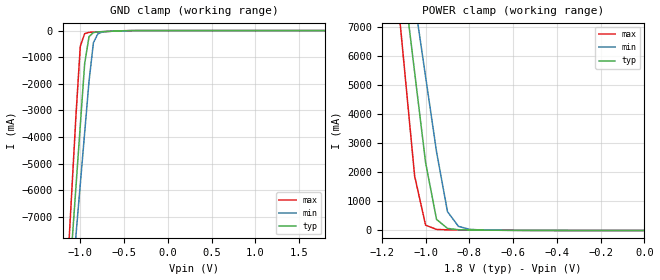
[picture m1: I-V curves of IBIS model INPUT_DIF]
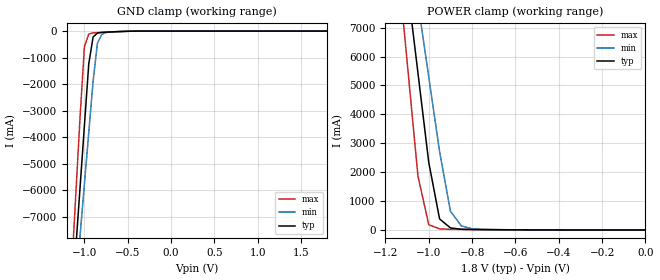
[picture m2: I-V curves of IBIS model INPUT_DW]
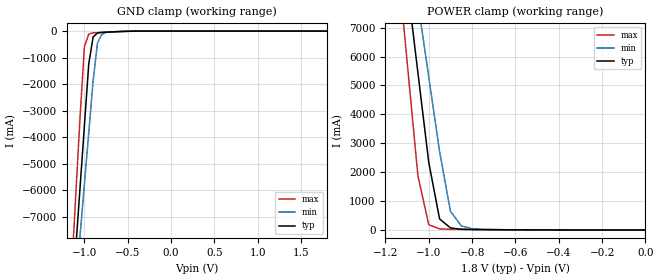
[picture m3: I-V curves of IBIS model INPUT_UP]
|   DIODES INCORPORATED
|   IBIS Model of PI6CB18801
|   Product Family: 6CB
|   TQFN 48-Pins (ZL) Package
[IBIS Ver] 3.2
[Comment char] |_char
[File Name] pi6cb18801_zl_reva.ibs
[File Rev] 1.0
[Source] File originated at Diodes Incorporated.
[Date] 12/18/18
[Disclaimer] (C) Copyright DIODES INCORPORATED
   All rights reserved
  Diodes Incorporated hereby grants the user of
  this IBIS model a non-exclusive, nontransferable license to
  use this IBIS model under the following terms.
  This IBIS model is provided on an "AS IS" basis and Diodes
  makes absolutely no warranty with respect to the information
  contained herein. DIODES DISCLAIMS AND CUSTOMER WAIVES ALL
  WARRANTIES, EXPRESSED OR IMPLIED, INCLUDING WARRANTIES OF
  MERCHANTABILITY OR FITNESS FOR A PARTICULAR PURPOSE. The
  entire risk as to quality and performance is with the customer.
  Accordingly, in no event shall the company be liable for any
  damages, whether in contract or tort, including any lost
  profits or other incidental, consequential, exemplary, or
  punitive damages arising out of the use or application of the
  IBIS model provided in this package. Further, Diodes reserves
  the right to make changes without notice to any product herein
  to improve reliability, function, or design. Diodes does not
  convey any license under patent rights or any other intellectual
  property rights, including those of third parties.
  The user is granted this license only to use the IBIS model
  and is not granted rights to sell, load, rent, lease or license
  the IBIS model in whole or in part, or in modified form to anyone
  other than user. User may modify the IBIS model to suit its specific
  application but rights to derivative works and such modifications
  shall belong to Diodes.
  Diodes is not obligated to provide maintenance or support
  for the licensed IBIS model.
  Contact Diodes at ATTN: APPLICATION ENGINEERING / IBIS MODELS
  1545 Barber Ln. Milpitas, CA 95035
[Component] PI6CB18801
[Manufacturer] Diodes Incorporated.
[Package]
| Variable   typ   min   max
R_pkg   0.03902ohm   0.02922ohm   0.04882ohm
L_pkg   0.79998nH   0.76828nH   0.83168nH
C_pkg   0.19606pF   0.17176pF   0.22036pF
[Pin]  signal_name   model_name   R_pin   L_pin   C_pin
1   SADR_TRI   INPUT_DW   0.04882   0.83168nH   0.22036pF
2   BW_SEL_TRI   NC   0.04490   0.81900nH   0.21064pF
3   NC   NC   0.04098   0.80632nH   0.20092pF
4   NC   NC   0.03706   0.79364nH   0.19120pF
5   VDD_R   POWER   0.03314   0.78096nH   0.18148pF
6   IN+   INPUT_DIF   0.02922   0.76828nH   0.17176pF
7   IN-   INPUT_DIF   0.02922   0.76828nH   0.17176pF
8   GND_R   GND   0.03314   0.78096nH   0.18148pF
9   GND_DIG   GND   0.03706   0.79364nH   0.19120pF
10   SCLK   INPUT_SCLK   0.04098   0.80632nH   0.20092pF
11   SDATA   IO   0.04490   0.81900nH   0.21064pF
12   VDD_DIG   POWER   0.04882   0.83168nH   0.22036pF
13   VDDO   POWER   0.04882   0.83168nH   0.22036pF
14   OE0#   INPUT_DW   0.04490   0.81900nH   0.21064pF
15   Q0+   HCSL_OUT   0.04098   0.80632nH   0.20092pF
16   Q0-   HCSL_OUT   0.03706   0.79364nH   0.19120pF
17   OE1#   INPUT_DW   0.03314   0.78096nH   0.18148pF
18   Q1+   HCSL_OUT   0.02922   0.76828nH   0.17176pF
19   Q1-   HCSL_OUT   0.02922   0.76828nH   0.17176pF
20   VDD   POWER   0.03314   0.78096nH   0.18148pF
21   VDDO   POWER   0.03706   0.79364nH   0.19120pF
22   GND   GND   0.04098   0.80632nH   0.20092pF
23   Q2+   HCSL_OUT   0.04490   0.81900nH   0.21064pF
24   Q2-   HCSL_OUT   0.04882   0.83168nH   0.22036pF
25   OE2#   INPUT_DW   0.04882   0.83168nH   0.22036pF
26   Q3+   HCSL_OUT   0.04490   0.81900nH   0.21064pF
27   Q3-   HCSL_OUT   0.04098   0.80632nH   0.20092pF
28   OE3#   INPUT_DW   0.03706   0.79364nH   0.19120pF
29   GNDA   GND   0.03314   0.78096nH   0.18148pF
30   VDDA   POWER   0.02922   0.76828nH   0.17176pF
31   VDDO   POWER   0.02922   0.76828nH   0.17176pF
32   Q4+   HCSL_OUT   0.03314   0.78096nH   0.18148pF
33   Q4-   HCSL_OUT   0.03706   0.79364nH   0.19120pF
34   OE4#   INPUT_DW   0.04098   0.80632nH   0.20092pF
35   Q5+   HCSL_OUT   0.04490   0.81900nH   0.21064pF
36   Q5-   HCSL_OUT   0.04882   0.83168nH   0.22036pF
37   OE5#   INPUT_DW   0.04882   0.83168nH   0.22036pF
38   VDD   POWER   0.04490   0.81900nH   0.21064pF
39   VDDO   POWER   0.04098   0.80632nH   0.20092pF
40   GND   GND   0.03706   0.79364nH   0.19120pF
41   Q6+   HCSL_OUT   0.03314   0.78096nH   0.18148pF
42   Q6-   HCSL_OUT   0.02922   0.76828nH   0.17176pF
43   OE6#   INPUT_DW   0.02922   0.76828nH   0.17176pF
44   Q7+   HCSL_OUT   0.03314   0.78096nH   0.18148pF
45   Q7-   HCSL_OUT   0.03706   0.79364nH   0.19120pF
46   OE7#   INPUT_DW   0.04098   0.80632nH   0.20092pF
47   VDDO   POWER   0.04490   0.81900nH   0.21064pF
48   PD#   INPUT_UP   0.04882   0.83168nH   0.22036pF
[Diff Pin] inv_pin vdiff  tdelay_typ tdelay_min tdelay_max
15   16   NA   NA   NA   NA
18   19   NA   NA   NA   NA
23   24   NA   NA   NA   NA
26   27   NA   NA   NA   NA
32   33   NA   NA   NA   NA
35   36   NA   NA   NA   NA
41   42   NA   NA   NA   NA
44   45   NA   NA   NA   NA
[Model selector] HCSL_OUT
HCSL_0P6_SLOW  Diff Output,Amplitude=0.6V,SMBUS=2v/ns,slow,slew_rate=0
HCSL_0P6_FAST  Diff Output,Amplitude=0.6V,SMBUS=3v/ns,fast,slew_rate=1
HCSL_0P7_SLOW  Diff Output,Amplitude=0.7V,SMBUS=2v/ns,slow,slew_rate=0
HCSL_0P7_FAST  Diff Output,Amplitude=0.7V,SMBUS=3v/ns,fast,slew_rate=1
HCSL_0P8_SLOW  Diff Output,Amplitude=0.8V,SMBUS=2v/ns,slow,slew_rate=0
HCSL_0P8_FAST  Diff Output,Amplitude=0.8V,SMBUS=3v/ns,fast,slew_rate=1
HCSL_0P9_SLOW  Diff Output,Amplitude=0.9V,SMBUS=2v/ns,slow,slew_rate=0
HCSL_0P9_FAST  Diff Output,Amplitude=0.9V,SMBUS=3v/ns,fast,slew_rate=1
| Models and submodels in the file (13): INPUT_DIF (Input), INPUT_DW (Input), INPUT_UP (Input), INPUT_SCLK (Input), IO (I/O_open_drain), HCSL_0P6_FAST (Output), HCSL_0P6_SLOW (Output), HCSL_0P7_FAST (Output), HCSL_0P7_SLOW (Output), HCSL_0P8_FAST (Output), HCSL_0P8_SLOW (Output), HCSL_0P9_FAST (Output), HCSL_0P9_SLOW (Output)
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|   Model INPUT_DIF
[Model] INPUT_DIF
Model_type Input
Vinl = 540.00mV
Vinh = 1.2600V
| variable   typ   min   max
C_comp   1.000pF   0.997pF   2.003pF
[Voltage Range]   1.8000V   1.7000V   1.9000V
[POWER Clamp Reference]   1.8000V   1.7000V   1.9000V
[GND Clamp Reference]   0.0000V   0.0000V   0.0000V
[Temperature Range]   25   85   -40
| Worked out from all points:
|   GND clamp passes 1 mA (typ) near -0.38 V on its own axis
|   POWER clamp passes 1 mA (typ) near -0.45 V on its own axis
[GND Clamp]
| Voltage   I(typ)   I(min)   I(max)
-1.8V     -40.8A     -36.77A    -47.86A
-1.15V    -10.55A    -11.59A    -9.184A
-1.1V     -8.222A    -9.649A    -6.209A
-1.05V    -5.896A    -7.712A    -3.234A
-1V       -3.569A    -5.775A    -591.1mA
-950mV    -1.243A    -3.838A    -113.6mA
-900mV    -226.2mA   -1.902A    -67.1mA
-850mV    -74.81mA   -458.6mA   -57.3mA
-800mV    -48.92mA   -124.4mA   -50.76mA
-750mV    -40.1mA    -53.68mA   -43.2mA
-350mV    -370.5uA   -927.1uA   -74.54uA
1.8V      1.6nA      277.6nA    24.82pA
[POWER Clamp]
| Voltage   I(typ)   I(min)   I(max)
-1.8V     52A        46.64A     61.4A
-1.15V    11.65A     13.04A     9.805A
-1.1V     8.543A     10.46A     5.838A
-1.05V    5.441A     7.877A     1.87A
-1V       2.338A     5.294A     182.4mA
-950mV    382.2mA    2.711A     36.45mA
-900mV    71.6mA     649.3mA    21.67mA
-850mV    24.87mA    142.8mA    18.04mA
-800mV    16.12mA    40.15mA    15.3mA
-750mV    12.63mA    17.74mA    12.39mA
0V        1.6nA      43.78nA    28.91pA
|   Model INPUT_DW
[Model] INPUT_DW
Model_type Input
Vinl = 540.00mV
Vinh = 1.2600V
| variable   typ   min   max
C_comp   1.000pF   0.997pF   2.003pF
[Voltage Range]   1.8000V   1.7000V   1.9000V
[POWER Clamp Reference]   1.8000V   1.7000V   1.9000V
[GND Clamp Reference]   0.0000V   0.0000V   0.0000V
[Temperature Range]   25   85   -40
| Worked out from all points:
|   GND clamp passes 1 mA (typ) near -0.38 V on its own axis
|   POWER clamp passes 1 mA (typ) near -0.45 V on its own axis
[GND Clamp]
| Voltage   I(typ)   I(min)   I(max)
-1.8V     -40.8A     -36.77A    -47.86A
-1.15V    -10.55A    -11.59A    -9.184A
-1.1V     -8.222A    -9.649A    -6.209A
-1.05V    -5.896A    -7.712A    -3.234A
-1V       -3.569A    -5.775A    -591.1mA
-950mV    -1.243A    -3.838A    -113.6mA
-900mV    -226.2mA   -1.902A    -67.1mA
-850mV    -74.82mA   -458.6mA   -57.31mA
-800mV    -48.93mA   -124.4mA   -50.76mA
-750mV    -40.11mA   -53.69mA   -43.2mA
-350mV    -373.5uA   -930.2uA   -77.22uA
1.8V      14.98uA    16.02uA    13.77uA
[POWER Clamp]
| Voltage   I(typ)   I(min)   I(max)
-1.8V     52A        46.64A     61.4A
-1.15V    11.65A     13.04A     9.805A
-1.1V     8.543A     10.46A     5.838A
-1.05V    5.441A     7.877A     1.87A
-1V       2.338A     5.294A     182.5mA
-950mV    382.2mA    2.711A     36.48mA
-900mV    71.62mA    649.3mA    21.69mA
-850mV    24.89mA    142.9mA    18.06mA
-800mV    16.15mA    40.17mA    15.32mA
-750mV    12.65mA    17.76mA    12.41mA
0V        14.98uA    14.91uA    14.54uA
|   Model INPUT_UP
[Model] INPUT_UP
Model_type Input
Vinl = 540.00mV
Vinh = 1.2600V
| variable   typ   min   max
C_comp   1.000pF   0.997pF   2.003pF
[Voltage Range]   1.8000V   1.7000V   1.9000V
[POWER Clamp Reference]   1.8000V   1.7000V   1.9000V
[GND Clamp Reference]   0.0000V   0.0000V   0.0000V
[Temperature Range]   25   85   -40
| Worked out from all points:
|   GND clamp passes 1 mA (typ) near -0.38 V on its own axis
|   POWER clamp passes 1 mA (typ) near -0.45 V on its own axis
[GND Clamp]
| Voltage   I(typ)   I(min)   I(max)
-1.8V     -40.8A     -36.77A    -47.86A
-1.15V    -10.55A    -11.59A    -9.184A
-1.1V     -8.222A    -9.649A    -6.209A
-1.05V    -5.896A    -7.712A    -3.234A
-1V       -3.569A    -5.775A    -591.1mA
-950mV    -1.243A    -3.838A    -113.7mA
-900mV    -226.2mA   -1.902A    -67.12mA
-850mV    -74.83mA   -458.6mA   -57.32mA
-800mV    -48.94mA   -124.4mA   -50.78mA
-750mV    -40.12mA   -53.71mA   -43.22mA
-350mV    -388.4uA   -945.1uA   -91.75uA
1.8V      1.6nA      1.152uA    -765nA
[POWER Clamp]
| Voltage   I(typ)   I(min)   I(max)
-1.8V     52A        46.64A     61.4A
-1.15V    11.65A     13.04A     9.805A
-1.1V     8.543A     10.46A     5.838A
-1.05V    5.441A     7.877A     1.87A
-1V       2.338A     5.294A     182.4mA
-950mV    382.2mA    2.711A     36.46mA
-900mV    71.6mA     649.3mA    21.68mA
-850mV    24.88mA    142.8mA    18.05mA
-800mV    16.13mA    40.15mA    15.31mA
-750mV    12.64mA    17.75mA    12.39mA
0V        1.6nA      43.78nA    28.91pA
